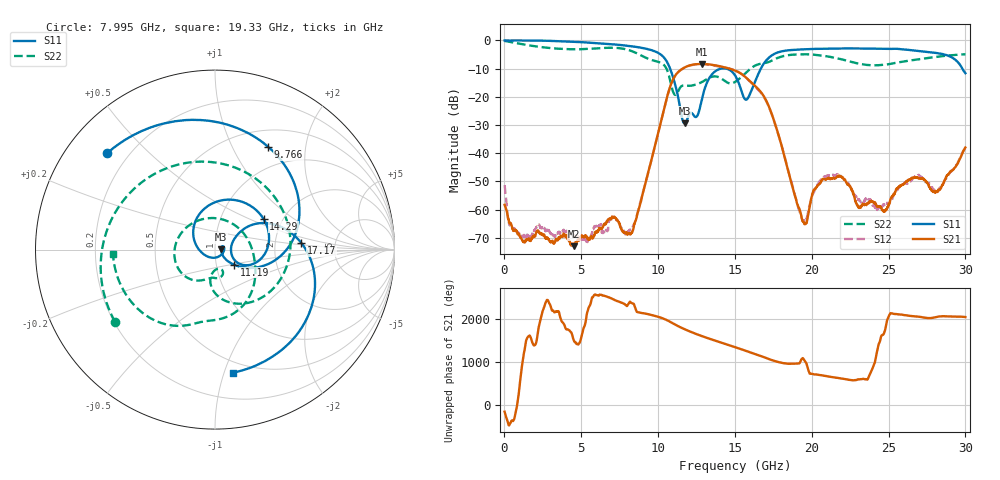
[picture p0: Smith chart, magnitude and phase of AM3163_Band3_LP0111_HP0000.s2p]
!Agilent Technologies,E8364B,MY43040894,A.07.50.67
!Agilent E8364B: A.07.50.67
!Date: Thursday, August 20, 2020 12:14:29
!Correction: S11(Full 2 Port(1,2))
!S21(Full 2 Port(1,2))
!S12(Full 2 Port(1,2))
!S22(Full 2 Port(1,2))
!S2P File: Measurements: S11, S21, S12, S22:
# Hz S  dB  R 50
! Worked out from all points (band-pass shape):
!   3201 points, 10 MHz to 30 GHz, reference 50 ohm
!   highest |S21| = -8.32 dB at 12.85 GHz (marker M1); lowest = -73.0 dB at 4.518 GHz (marker M2)
!   |S21| within 3 dB of the highest: 11.29 GHz to 15.26 GHz (3.974 GHz wide, 29.9 % of centre)
!   lowest |S11| = -29.5 dB at 11.72 GHz (marker M3), VSWR 1.07, Z = 53.5 + j0.194 ohm
!   |S11| at or under -10 dB: 10.78 GHz to 14.09 GHz (3.311 GHz wide, 26.6 % of centre); 14.44 GHz to 16.69 GHz (2.241 GHz wide, 14.4 % of centre); 29.8 GHz to end of sweep
!   |S22| runs from -19.3 to -0.2 dB; largest |S21 - S12| = 0.0089
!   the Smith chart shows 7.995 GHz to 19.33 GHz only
!   S11 on the Smith chart (normalised r, x): 7.995 GHz: 0.12, +0.38; 9.766 GHz: 0.71, +1.39; 11.19 GHz: 1.22, -0.21; 14.29 GHz: 1.60, +0.61; 17.17 GHz: 2.84, +0.27; 19.33 GHz: 0.41, -1.07
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1e7  -0.01 -1.9  -58.30 -143.3  -51.33 108.5  -0.21 -5.9
1.040906e9  -0.00 -28.5  -69.96 -85.7  -69.02 -72.6  -1.23 -81.9
2.296738e9  -0.07 -63.0  -68.25 105.6  -65.84 -127.5  -2.28 -161.0
4.517872e9  -0.47 -122.4  -72.97 62.6  -69.13 78.7  -3.13 81.0
5.014581e9  -0.61 -135.6  -69.27 152.9  -70.53 76.7  -3.10 54.1
6.354759e9  -1.06 -172.1  -66.61 26.8  -68.04 25.4  -2.70 -25.0
7.994838e9  -1.87 138.1  -68.88 144.7  -68.27 118.0  -3.26 -144.3
8.997628e9  -2.67 100.4  -54.36 -28.4  -54.16 -26.3  -5.59 119.4
9.766122e9  -3.81 62.6  -38.03 -88.2  -38.05 -89.0  -7.21 29.8
1.000979e10  -4.43 47.6  -32.68 -112.7  -32.75 -113.8  -7.56 -0.7
1.119065e10  -17.38 -38.4  -11.91 52.1  -11.95 52.3  -19.12 -75.2
1.172484e10  -29.45 3.1  -9.59 -39.2  -9.65 -39.3  -15.94 -86.3
1.284947e10  -20.81 178.5  -8.32 162.0  -8.39 161.9  -14.76 -111.7
1.429274e10  -9.90 32.3  -9.49 -9.6  -9.55 -8.3  -14.18 133.6
1.5005e10  -12.35 -17.2  -10.67 -92.0  -10.61 -91.6  -14.72 29.1
1.576412e10  -20.94 5.1  -13.37 176.0  -13.45 175.6  -11.22 -35.9
1.71699e10  -6.33 4.3  -22.89 -3.0  -23.10 -0.9  -7.70 -101.4
1.932543e10  -3.19 -81.5  -62.40 -16.0  -62.60 -73.8  -4.90 -177.3
2.000958e10  -3.02 -100.0  -55.13 11.0  -55.36 -81.5  -5.00 158.0
2.298984e10  -2.85 -168.4  -58.62 -120.9  -56.38 -150.8  -8.15 25.6
2.500479e10  -3.00 144.2  -58.16 -106.5  -57.72 -138.3  -8.42 -82.3
3e10  -11.61 -28.4  -37.99 -118.3  -38.45 -121.6  -4.91 103.2
